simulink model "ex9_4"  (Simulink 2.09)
settings: Solver=ode23s  StartTime=0.0  StopTime=1000.0  MaxStep=.1  RelTol=1e-3  AbsTol=1e-6
undefined symbols (not defined in the file or in its folder): start_sim, stop_sim, strtstpm

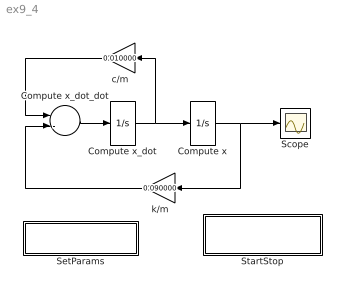
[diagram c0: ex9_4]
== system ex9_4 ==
  Compute x : Integrator  ExternalReset=none  InitialConditionSource=internal  InitialCondition=0  LimitOutput=off  UpperSaturationLimit=inf  LowerSaturationLimit=-inf  ShowSaturationPort=off  ShowStatePort=off  AbsoluteTolerance=auto
  Compute x_dot : Integrator  ExternalReset=none  InitialConditionSource=internal  InitialCondition=1  LimitOutput=off  UpperSaturationLimit=inf  LowerSaturationLimit=-inf  ShowSaturationPort=off  ShowStatePort=off  AbsoluteTolerance=auto
  Compute x_dot_dot : Sum  Inputs=--
  Scope : Scope
  SetParams : Subsystem  mask{m=1.000000, c=0.010000, k=0.090000}
      mask prompts: m "Mass"; c "Damping coefficient"; k "Spring constant"
      mask help: This masked subsystem supports the spring-mass user interface. The dialog fiellds are not available to the user due to the use of the OperFcn callback.
  StartStop : Subsystem  StartFcn=strtstpm start_sim  StopFcn=strtstpm stop_sim
  c/m : Gain  Orientation=left  Gain=0.010000
  k/m : Gain  Orientation=left  Gain=0.090000
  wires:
  Compute x_dot_dot/1 -> Compute x_dot/1
  c/m/1 -> Compute x_dot_dot/1
  Compute x_dot/1 -> Compute x/1, c/m/1
  k/m/1 -> Compute x_dot_dot/2
  Compute x/1 -> k/m/1, Scope/1

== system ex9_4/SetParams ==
  note: This is an empty subsystem. The purpose of the subsystem is to provide a means to open the sys_set user interface.

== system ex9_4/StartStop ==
  note: This is an empty subsystem. The purpose of the subsystem is to provide a means to open the sys_set user interface.
